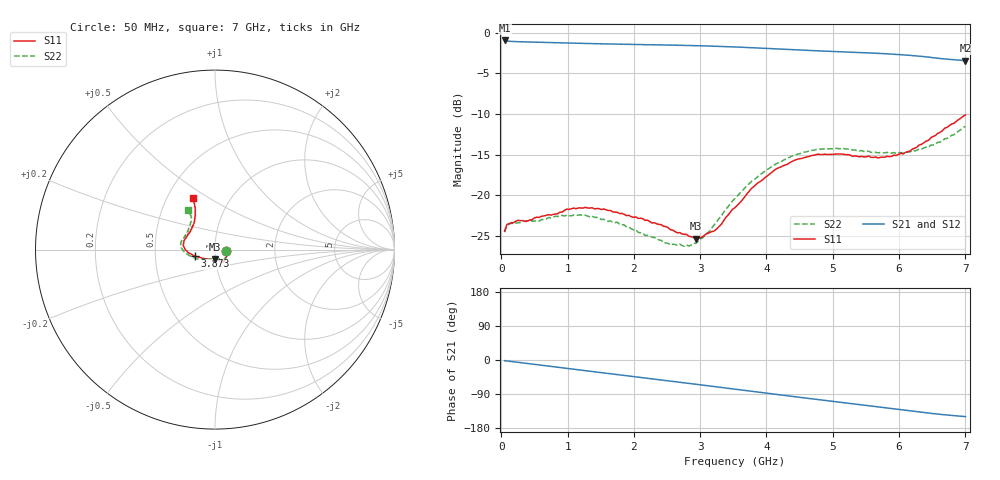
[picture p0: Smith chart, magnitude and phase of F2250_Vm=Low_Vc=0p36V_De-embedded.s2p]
! Integrated Device Technology
! Corporate Headquarters
! 6024 Silver Creek Valley Road
! San Jose, CA 95138  USA
! Phone:  1-408-284-8200
! Toll Free:  1-800-223-1366
! Webpage:  http://www.idt.com/
! Timing and RF Division
! 515 Groton Road, Suite 102
! Westford, MA 01886-6024
! Device:  F2250
! Description: Voltage Variable RF Attenuator
! Frequency:  50.0 -  6000.00 MHz
! Package:  3x3 mm Thin QFN Plastic Package: 16 pin
! Ports:  2 RF, 3 DC
!  Pin  1  = GND
!  Pin  2  = NC
!  Pin  3  = RF1  = Port 1
!  Pin  4  = NC
!  Pin  5  = GND
!  Pin  6  = GND
!  Pin  7  = GND
!  Pin  8  = GND
!  Pin  9  = NC
!  Pin 10  = RF2  = Port 2
!  Pin 11  = NC
!  Pin 12  = GND
!  Pin 13  = GND
!  Pin 14  = VCNTRL
!  Pin 15  = VDD
!  Pin 16  = VMODE
! Vcntrl:  0.360 Volts
! Vmode:  +0.000 Volts
! Vdd:  +3.30  Volts
! Current:  1.119 mA
! Data:  The device was measured on a the F2250 evaluation board which has
!  individual transmission lines to the RF pins.  Data was collected
!  using a calibrated network analyzer.  The evaluation board was
!  de-embedded using a TRL calibration technique.
!  The reference plane is the edge of the package pin.
! Misc:  SN 10
!  Action Tracker AT0258
! Date Measured:  2014-11-26
! Date:  2015-10-15  MJV
! Note:
!  Integrated Device Technology supplies this data as a sample of measured
!  data at the package pin for this product.  Your particular data for this
!  product may vary.
!  Data was taken at 25 degrees C.
!  Integrated Device Technology reserves the right to change this data at anytime.
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# GHz S dB R 50
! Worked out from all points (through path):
!   201 points, 50 MHz to 7 GHz, reference 50 ohm
!   highest |S21| = -0.97 dB at 50 MHz (marker M1); lowest = -3.5 dB at 7 GHz (marker M2)
!   group delay of S21, straight-line fit = 60 ps
!   lowest |S11| = -25.3 dB at 2.934 GHz (marker M3), VSWR 1.11, Z = 49.9 - j5.41 ohm
!   |S11| at or under -10 dB: start of sweep to end of sweep
!   |S22| runs from -26.2 to -11.5 dB; largest |S21 - S12| = 0.00033
!   S11 on the Smith chart (normalised r, x): 50 MHz: 1.13, -0.02; 3.873 GHz: 0.79, -0.06; 7 GHz: 0.67, +0.42
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0.05  -24.39 -9.0  -0.97 -1.8  -0.97 -1.8  -24.53 -9.6
0.08475  -23.58 -9.0  -1.05 -2.5  -1.04 -2.5  -23.67 -8.9
0.15425  -23.36 -11.2  -1.09 -4.0  -1.09 -4.0  -23.44 -10.6
0.6755  -22.47 -34.4  -1.22 -15.4  -1.21 -15.4  -22.91 -35.4
0.98825  -21.69 -48.1  -1.28 -22.2  -1.28 -22.2  -22.42 -51.1
1.2315  -21.58 -53.8  -1.33 -27.4  -1.33 -27.4  -22.48 -58.4
1.75275  -22.10 -60.5  -1.43 -38.4  -1.42 -38.4  -23.31 -66.0
2.37825  -23.58 -61.6  -1.52 -51.8  -1.51 -51.8  -25.48 -68.8
2.552  -24.22 -65.5  -1.54 -55.6  -1.54 -55.6  -26.12 -74.5
2.83  -25.03 -79.9  -1.59 -61.7  -1.59 -61.7  -26.23 -92.9
2.93425  -25.34 -88.4  -1.61 -64.0  -1.61 -64.0  -25.90 -101.3
3.21225  -24.38 -117.4  -1.68 -70.2  -1.68 -70.2  -23.63 -126.5
3.525  -21.51 -144.9  -1.77 -77.1  -1.77 -77.1  -20.40 -145.4
3.8725  -18.46 -161.9  -1.90 -84.8  -1.90 -84.8  -17.68 -160.8
4.1505  -16.74 -171.9  -2.02 -90.9  -2.01 -90.9  -16.11 -170.8
4.4285  -15.69 -179.6  -2.12 -96.9  -2.12 -96.9  -15.03 -178.0
4.7065  -15.08 173.6  -2.23 -102.9  -2.23 -102.9  -14.47 176.0
5.15825  -14.95 162.8  -2.38 -112.6  -2.38 -112.6  -14.23 166.8
5.85325  -15.25 139.6  -2.63 -127.5  -2.63 -127.6  -14.84 151.6
6.166  -14.56 128.5  -2.80 -134.4  -2.80 -134.4  -14.66 142.7
6.444  -13.24 120.1  -3.01 -140.1  -3.01 -140.2  -14.06 133.3
7  -10.13 113.5  -3.45 -149.4  -3.45 -149.4  -11.53 123.9
